FUNCTION_BLOCK FB 24
TITLE =
AUTHOR : WE_ZA
FAMILY : Ablauf
NAME : BETR
VERSION : 0.1


VAR_INPUT
  STG_AUS : BOOL ;
  STG_EIN : BOOL ;
  START : BOOL ;
  AUTO : BOOL ;
  EmB : BOOL ;
  EoB : BOOL ;
  EINR : BOOL ;
  ZYKLUS : BOOL ;
  NOT_AUS : BOOL ;
  AKTOR_FR : BOOL ;
  GST_ANL : BOOL ;
  SCHRITT : INT ;
END_VAR
VAR_OUTPUT
  ANZ_STG : BOOL ;
  ANZ_AUTO : BOOL ;
  ANZ_EmB : BOOL ;
  ANZ_EoB : BOOL ;
  ANZ_EINR : BOOL ;
  ANZ_ZYK_E : BOOL ;
  ANZ_ZYK_A : BOOL ;
  RESET : BOOL ;
  FR_K_mB : BOOL ;
  FR_K_oB : BOOL ;
  FR_AKTION : BOOL ;
END_VAR
VAR
  STEU_EIN : BOOL ;
  AUTO_EIN : BOOL ;
  AUTO_BE : BOOL ;
  START_SP : BOOL ;
  FO1 : BOOL ;
  FO2 : BOOL ;
  IO_WEITER : BOOL ;
END_VAR
BEGIN
NETWORK
TITLE =
//Steuerung EIN-AUS
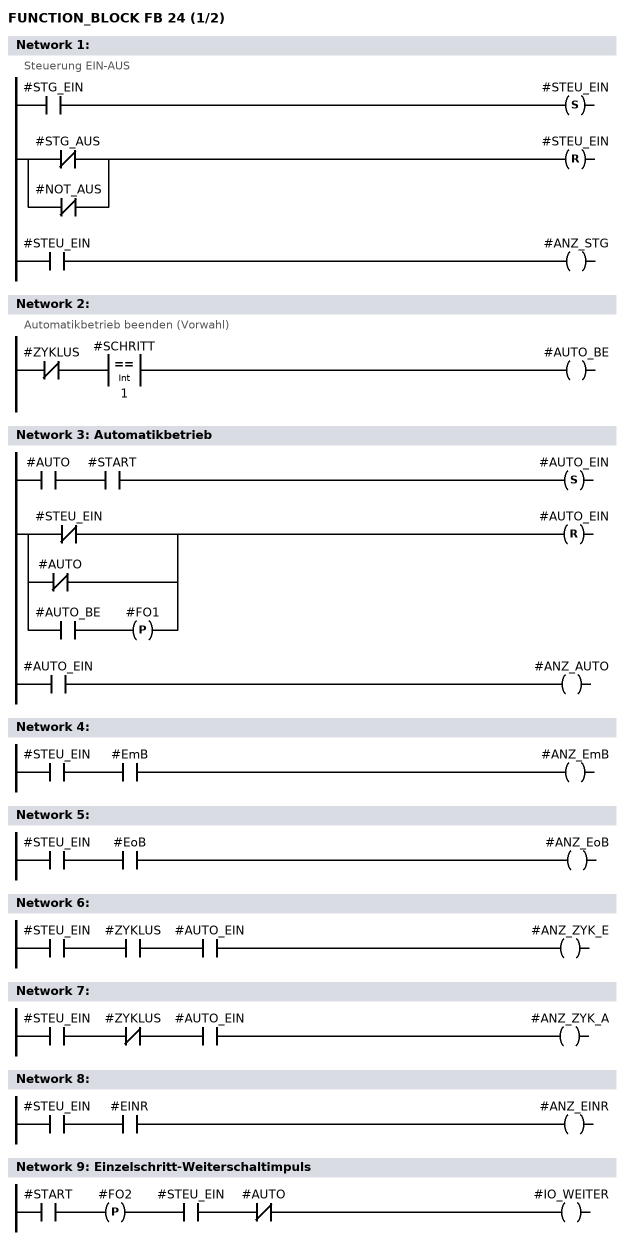
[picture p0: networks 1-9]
      U     #STG_EIN;
      S     #STEU_EIN;
      U(    ;
      ON    #STG_AUS;
      ON    #NOT_AUS;
      )     ;
      R     #STEU_EIN;
      U     #STEU_EIN;
      =     #ANZ_STG;
NETWORK
TITLE =
//Automatikbetrieb beenden (Vorwahl)
      UN    #ZYKLUS;
      U(    ;
      L     #SCHRITT;
      L     1;
      ==I   ;
      )     ;
      =     #AUTO_BE;
NETWORK
TITLE =Automatikbetrieb

      U     #AUTO;
      U     #START;
      S     #AUTO_EIN;
      U(    ;
      ON    #STEU_EIN;
      ON    #AUTO;
      O(    ;
      U     #AUTO_BE;
      FP    #FO1;
      )     ;
      )     ;
      R     #AUTO_EIN;
      U     #AUTO_EIN;
      =     #ANZ_AUTO;
NETWORK
TITLE =

      U     #STEU_EIN;
      U     #EmB;
      =     #ANZ_EmB;
NETWORK
TITLE =

      U     #STEU_EIN;
      U     #EoB;
      =     #ANZ_EoB;
NETWORK
TITLE =

      U     #STEU_EIN;
      U     #ZYKLUS;
      U     #AUTO_EIN;
      =     #ANZ_ZYK_E;
NETWORK
TITLE =

      U     #STEU_EIN;
      UN    #ZYKLUS;
      U     #AUTO_EIN;
      =     #ANZ_ZYK_A;
NETWORK
TITLE =

      U     #STEU_EIN;
      U     #EINR;
      =     #ANZ_EINR;
NETWORK
TITLE =Einzelschritt-Weiterschaltimpuls

      U     #START;
      FP    #FO2;
      U     #STEU_EIN;
      UN    #AUTO;
      =     #IO_WEITER;
NETWORK
TITLE =Freigabe Kette mit Bedingungen
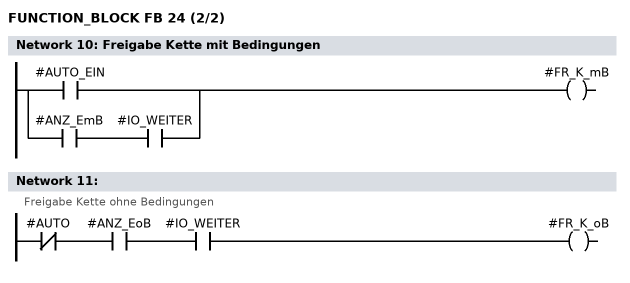
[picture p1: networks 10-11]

      O     #AUTO_EIN;
      O     ;
      U     #ANZ_EmB;
      U     #IO_WEITER;
      =     #FR_K_mB;
NETWORK
TITLE =
//Freigabe Kette ohne Bedingungen
      UN    #AUTO;
      U     #ANZ_EoB;
      U     #IO_WEITER;
      =     #FR_K_oB;
NETWORK
TITLE =Aktionsfreigabe

      U(    ;
      O     #AUTO_EIN;
      O     ;
      U     #ANZ_EmB;
      U(    ;
      U     #START;
      S     #START_SP;
      UN    #STEU_EIN;
      R     #START_SP;
      U     #START_SP;
      )     ;
      O     ;
      U     #ANZ_EoB;
      U     #AKTOR_FR;
      )     ;
      U     #STEU_EIN;
      =     #FR_AKTION;
NETWORK
TITLE =Rücksetzen Schrittkette u.a.
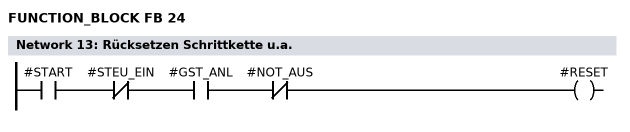
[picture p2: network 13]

      U     #START;
      UN    #STEU_EIN;
      U     #GST_ANL;
      UN    #NOT_AUS;
      =     #RESET;
END_FUNCTION_BLOCK

FUNCTION_BLOCK FB 25
TITLE =
AUTHOR : WE_ZA
FAMILY : Ablauf
NAME : KET_10
VERSION : 0.1


VAR_INPUT
  RESET : BOOL ;
  WEITER_mB : BOOL ;
  WEITER_oB : BOOL ;
  T1_2 : BOOL ;
  T2_3 : BOOL  := TRUE;
  T3_4 : BOOL  := TRUE;
  T4_5 : BOOL  := TRUE;
  T5_6 : BOOL  := TRUE;
  T6_7 : BOOL  := TRUE;
  T7_8 : BOOL  := TRUE;
  T8_9 : BOOL  := TRUE;
  T9_10 : BOOL  := TRUE;
  T10_1 : BOOL  := TRUE;
END_VAR
VAR_OUTPUT
  SCHRITT : INT ;
END_VAR
VAR
  SRO_1 : BOOL  := TRUE;
  SRO_2 : BOOL ;
  SRO_3 : BOOL ;
  SRO_4 : BOOL ;
  SRO_5 : BOOL ;
  SRO_6 : BOOL ;
  SRO_7 : BOOL ;
  SRO_8 : BOOL ;
  SRO_9 : BOOL ;
  SRO_10 : BOOL ;
END_VAR
BEGIN
NETWORK
TITLE =



      U(    ;
      U(    ;
      O     #RESET;
      O     ;
      UN    #SRO_9;
      U     #SRO_10;
      U(    ;
      U     #WEITER_mB;
      U     #T10_1;
      O     #WEITER_oB;
      )     ;
      )     ;
      S     #SRO_1;
      U     #SRO_2;
      R     #SRO_1;
      U     #SRO_1;
      )     ;
      SPBNB _001;
      L     1;
      T     #SCHRITT;
_001: NOP   0;
NETWORK
TITLE =

      U(    ;
      U     #SRO_1;
      UN    #SRO_10;
      U(    ;
      U     #WEITER_mB;
      U     #T1_2;
      O     #WEITER_oB;
      )     ;
      S     #SRO_2;
      U(    ;
      O     #RESET;
      O     #SRO_3;
      )     ;
      R     #SRO_2;
      U     #SRO_2;
      )     ;
      SPBNB _002;
      L     2;
      T     #SCHRITT;
_002: NOP   0;
NETWORK
TITLE =

      U(    ;
      U     #SRO_2;
      UN    #SRO_1;
      U(    ;
      U     #WEITER_mB;
      U     #T2_3;
      O     #WEITER_oB;
      )     ;
      S     #SRO_3;
      U(    ;
      O     #RESET;
      O     #SRO_4;
      )     ;
      R     #SRO_3;
      U     #SRO_3;
      )     ;
      SPBNB _003;
      L     3;
      T     #SCHRITT;
_003: NOP   0;
NETWORK
TITLE =

      U(    ;
      U     #SRO_3;
      UN    #SRO_2;
      U(    ;
      U     #WEITER_mB;
      U     #T3_4;
      O     #WEITER_oB;
      )     ;
      S     #SRO_4;
      U(    ;
      O     #RESET;
      O     #SRO_5;
      )     ;
      R     #SRO_4;
      U     #SRO_4;
      )     ;
      SPBNB _004;
      L     4;
      T     #SCHRITT;
_004: NOP   0;
NETWORK
TITLE =

      U(    ;
      U     #SRO_4;
      UN    #SRO_3;
      U(    ;
      U     #WEITER_mB;
      U     #T4_5;
      O     #WEITER_oB;
      )     ;
      S     #SRO_5;
      U(    ;
      O     #RESET;
      O     #SRO_6;
      )     ;
      R     #SRO_5;
      U     #SRO_5;
      )     ;
      SPBNB _005;
      L     5;
      T     #SCHRITT;
_005: NOP   0;
NETWORK
TITLE =

      U(    ;
      U     #SRO_5;
      UN    #SRO_4;
      U(    ;
      U     #WEITER_mB;
      U     #T5_6;
      O     #WEITER_oB;
      )     ;
      S     #SRO_6;
      U(    ;
      O     #RESET;
      O     #SRO_7;
      )     ;
      R     #SRO_6;
      U     #SRO_6;
      )     ;
      SPBNB _006;
      L     6;
      T     #SCHRITT;
_006: NOP   0;
NETWORK
TITLE =

      U(    ;
      U     #SRO_6;
      UN    #SRO_5;
      U(    ;
      U     #WEITER_mB;
      U     #T6_7;
      O     #WEITER_oB;
      )     ;
      S     #SRO_7;
      U(    ;
      O     #RESET;
      O     #SRO_8;
      )     ;
      R     #SRO_7;
      U     #SRO_7;
      )     ;
      SPBNB _007;
      L     7;
      T     #SCHRITT;
_007: NOP   0;
NETWORK
TITLE =

      U(    ;
      U     #SRO_7;
      UN    #SRO_6;
      U(    ;
      U     #WEITER_mB;
      U     #T7_8;
      O     #WEITER_oB;
      )     ;
      S     #SRO_8;
      U(    ;
      O     #RESET;
      O     #SRO_9;
      )     ;
      R     #SRO_8;
      U     #SRO_8;
      )     ;
      SPBNB _008;
      L     8;
      T     #SCHRITT;
_008: NOP   0;
NETWORK
TITLE =

      U(    ;
      U     #SRO_8;
      UN    #SRO_7;
      U(    ;
      U     #WEITER_mB;
      U     #T8_9;
      O     #WEITER_oB;
      )     ;
      S     #SRO_9;
      U(    ;
      O     #RESET;
      O     #SRO_10;
      )     ;
      R     #SRO_9;
      U     #SRO_9;
      )     ;
      SPBNB _009;
      L     9;
      T     #SCHRITT;
_009: NOP   0;
NETWORK
TITLE =

      U(    ;
      U     #SRO_9;
      UN    #SRO_8;
      U(    ;
      U     #WEITER_mB;
      U     #T9_10;
      O     #WEITER_oB;
      )     ;
      S     #SRO_10;
      U(    ;
      O     #RESET;
      O     #SRO_1;
      )     ;
      R     #SRO_10;
      U     #SRO_10;
      )     ;
      SPBNB _00a;
      L     10;
      T     #SCHRITT;
_00a: NOP   0;
END_FUNCTION_BLOCK

FUNCTION FC 26 : VOID
TITLE =
VERSION : 0.1


VAR_INPUT
  SCHRITT : INT ;
  FREIGABE : BOOL ;
  EINRI : BOOL ;
  RESET : BOOL ;
  A_ANW : BYTE ;
  A_AST : BOOL ;
  A_GST : BOOL ;
  _1B1 : BOOL ;
  _1B2 : BOOL ;
  _2B1 : BOOL ;
  _3B1 : BOOL ;
  S1 : BOOL ;
  S2 : BOOL ;
  S3 : BOOL ;
  Zeit_1 : TIMER ;
  Zeitw_1 : S5TIME ;
  Zeit_2 : TIMER ;
  Zeitw_2 : S5TIME ;
END_VAR
VAR_OUTPUT
  _1Y1 : BOOL ;
  _1Y2 : BOOL ;
  _2Y1 : BOOL ;
  _3Y1 : BOOL ;
  K1 : BOOL ;
  K2 : BOOL ;
END_VAR
VAR_TEMP
  Aktor : INT ;
END_VAR
BEGIN
NETWORK
TITLE =

      L     #A_ANW;
      L     B#16#F;
      UW    ;
      T     #Aktor;
NETWORK
TITLE =Ansteuerung 1Y1 Zylinder 1A vor
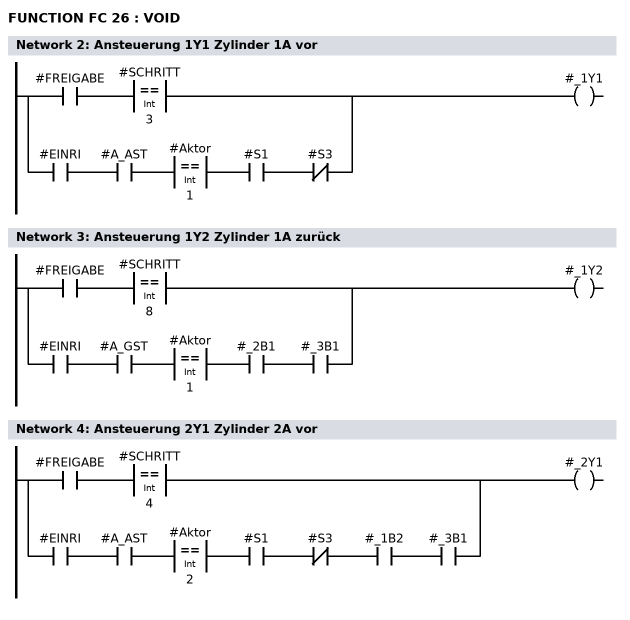
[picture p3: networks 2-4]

      U     #FREIGABE;
      U(    ;
      L     #SCHRITT;
      L     3;
      ==I   ;
      )     ;
      O     ;
      U     #EINRI;
      U     #A_AST;
      U(    ;
      L     #Aktor;
      L     1;
      ==I   ;
      )     ;
      U     #S1;
      UN    #S3;
      =     #_1Y1;
NETWORK
TITLE =Ansteuerung 1Y2 Zylinder 1A zurück

      U     #FREIGABE;
      U(    ;
      L     #SCHRITT;
      L     8;
      ==I   ;
      )     ;
      O     ;
      U     #EINRI;
      U     #A_GST;
      U(    ;
      L     #Aktor;
      L     1;
      ==I   ;
      )     ;
      U     #_2B1;
      U     #_3B1;
      =     #_1Y2;
NETWORK
TITLE =Ansteuerung 2Y1 Zylinder 2A vor

      U     #FREIGABE;
      U(    ;
      L     #SCHRITT;
      L     4;
      ==I   ;
      )     ;
      O     ;
      U     #EINRI;
      U     #A_AST;
      U(    ;
      L     #Aktor;
      L     2;
      ==I   ;
      )     ;
      U     #S1;
      UN    #S3;
      U     #_1B2;
      U     #_3B1;
      =     #_2Y1;
NETWORK
TITLE =Ansteuerung 2Y1 Zylinder 3A vor

      U     #FREIGABE;
      U(    ;
      O(    ;
      L     #SCHRITT;
      L     6;
      ==I   ;
      )     ;
      O(    ;
      U(    ;
      L     #SCHRITT;
      L     7;
      ==I   ;
      )     ;
      L     #Zeitw_1;
      SI    #Zeit_1;
      U(    ;
      O     #RESET;
      ON    #FREIGABE;
      )     ;
      R     #Zeit_1;
      NOP   0;
      NOP   0;
      U     #Zeit_1;
      )     ;
      )     ;
      O     ;
      U     #EINRI;
      U     #A_AST;
      U(    ;
      L     #Aktor;
      L     3;
      ==I   ;
      )     ;
      U     #S1;
      UN    #S3;
      U     #_1B2;
      U     #_2B1;
      =     #_3Y1;
NETWORK
TITLE = Ansteuerung K1 Schutztür zu

      U(    ;
      U     #FREIGABE;
      U(    ;
      U(    ;
      L     #SCHRITT;
      L     2;
      ==I   ;
      )     ;
      L     #Zeitw_2;
      SE    #Zeit_2;
      U(    ;
      O     #RESET;
      ON    #FREIGABE;
      )     ;
      R     #Zeit_2;
      NOP   0;
      NOP   0;
      U     #Zeit_2;
      )     ;
      O     ;
      U     #EINRI;
      U     #A_AST;
      U(    ;
      L     #Aktor;
      L     4;
      ==I   ;
      )     ;
      )     ;
      U     #S3;
      =     #K1;
NETWORK
TITLE =Ansteuerung K2 Schutztüre Auf
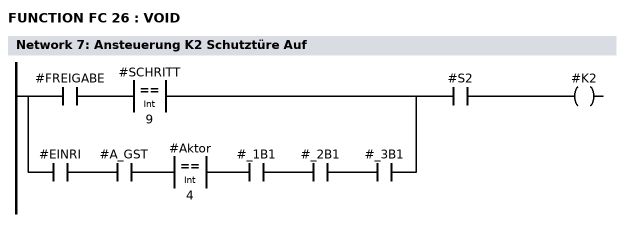
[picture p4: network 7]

      U(    ;
      U     #FREIGABE;
      U(    ;
      L     #SCHRITT;
      L     9;
      ==I   ;
      )     ;
      O     ;
      U     #EINRI;
      U     #A_GST;
      U(    ;
      L     #Aktor;
      L     4;
      ==I   ;
      )     ;
      U     #_1B1;
      U     #_2B1;
      U     #_3B1;
      )     ;
      U     #S2;
      =     #K2;
END_FUNCTION

ORGANIZATION_BLOCK OB 1
TITLE = "Main Program Sweep (Cycle)"
VERSION : 0.1


VAR_TEMP
  OB1_EV_CLASS : BYTE ;	//Bits 0-3 = 1 (Coming event), Bits 4-7 = 1 (Event class 1)
  OB1_SCAN_1 : BYTE ;	//1 (Cold restart scan 1 of OB 1), 3 (Scan 2-n of OB 1)
  OB1_PRIORITY : BYTE ;	//Priority of OB Execution
  OB1_OB_NUMBR : BYTE ;	//1 (Organization block 1, OB1)
  OB1_RESERVED_1 : BYTE ;	//Reserved for system
  OB1_RESERVED_2 : BYTE ;	//Reserved for system
  OB1_PREV_CYCLE : INT ;	//Cycle time of previous OB1 scan (milliseconds)
  OB1_MIN_CYCLE : INT ;	//Minimum cycle time of OB1 (milliseconds)
  OB1_MAX_CYCLE : INT ;	//Maximum cycle time of OB1 (milliseconds)
  OB1_DATE_TIME : DATE_AND_TIME ;	//Date and time OB1 started
  GA : BOOL ;
  Schritt : INT ;
  B0 : BOOL ;
  B1 : BOOL ;
  B2 : BOOL ;
  B3 : BOOL ;
END_VAR
BEGIN
NETWORK
TITLE =
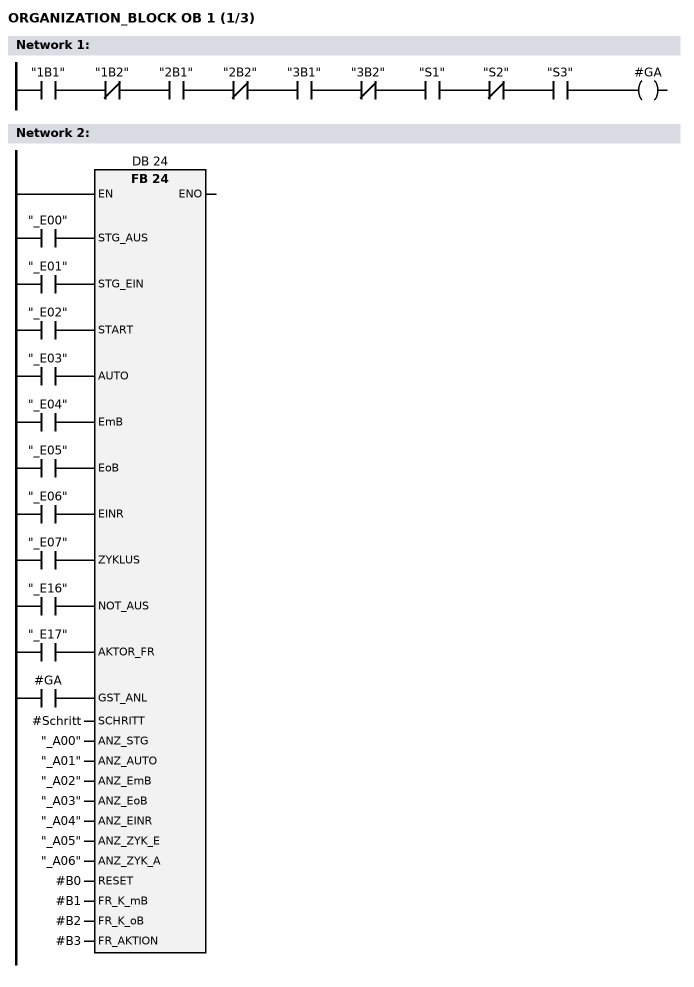
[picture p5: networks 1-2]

      U     "1B1";
      UN    "1B2";
      U     "2B1";
      UN    "2B2";
      U     "3B1";
      UN    "3B2";
      U     "S1";
      UN    "S2";
      U     "S3";
      =     #GA;
NETWORK
TITLE =

      U     "_E00";
      =     L     25.0;
      BLD   103;
      U     "_E01";
      =     L     25.1;
      BLD   103;
      U     "_E02";
      =     L     25.2;
      BLD   103;
      U     "_E03";
      =     L     25.3;
      BLD   103;
      U     "_E04";
      =     L     25.4;
      BLD   103;
      U     "_E05";
      =     L     25.5;
      BLD   103;
      U     "_E06";
      =     L     25.6;
      BLD   103;
      U     "_E07";
      =     L     25.7;
      BLD   103;
      U     "_E16";
      =     L     26.0;
      BLD   103;
      U     "_E17";
      =     L     26.1;
      BLD   103;
      U     #GA;
      =     L     26.2;
      BLD   103;
      CALL FB    24 , DB    24 (
           STG_AUS                  := L     25.0,
           STG_EIN                  := L     25.1,
           START                    := L     25.2,
           AUTO                     := L     25.3,
           EmB                      := L     25.4,
           EoB                      := L     25.5,
           EINR                     := L     25.6,
           ZYKLUS                   := L     25.7,
           NOT_AUS                  := L     26.0,
           AKTOR_FR                 := L     26.1,
           GST_ANL                  := L     26.2,
           SCHRITT                  := #Schritt,
           ANZ_STG                  := "_A00",
           ANZ_AUTO                 := "_A01",
           ANZ_EmB                  := "_A02",
           ANZ_EoB                  := "_A03",
           ANZ_EINR                 := "_A04",
           ANZ_ZYK_E                := "_A05",
           ANZ_ZYK_A                := "_A06",
           RESET                    := #B0,
           FR_K_mB                  := #B1,
           FR_K_oB                  := #B2,
           FR_AKTION                := #B3);
      NOP   0;
NETWORK
TITLE =
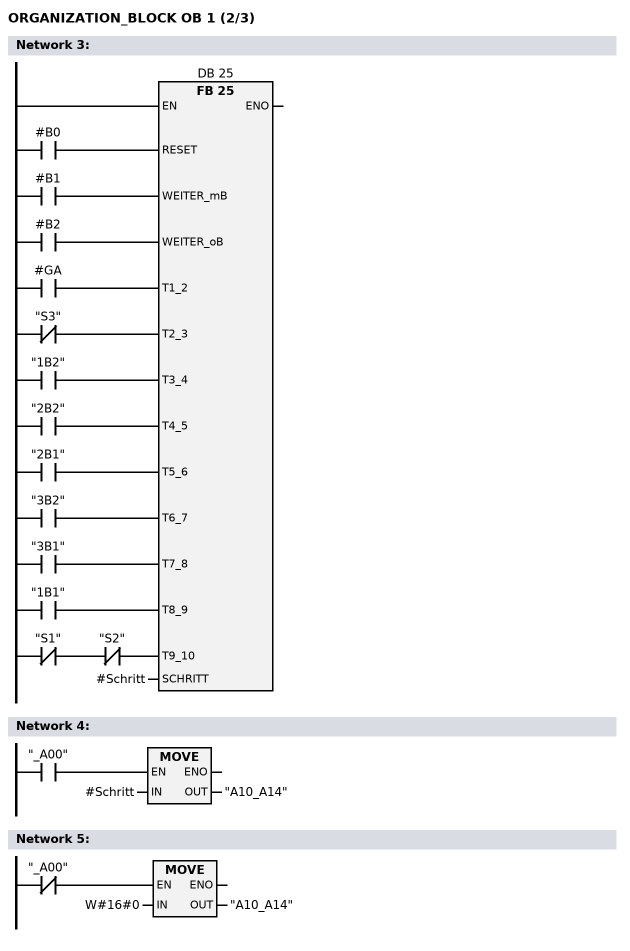
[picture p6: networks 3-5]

      U     #B0;
      =     L     25.0;
      BLD   103;
      U     #B1;
      =     L     25.1;
      BLD   103;
      U     #B2;
      =     L     25.2;
      BLD   103;
      U     #GA;
      =     L     25.3;
      BLD   103;
      UN    "S3";
      =     L     25.4;
      BLD   103;
      U     "1B2";
      =     L     25.5;
      BLD   103;
      U     "2B2";
      =     L     25.6;
      BLD   103;
      U     "2B1";
      =     L     25.7;
      BLD   103;
      U     "3B2";
      =     L     26.0;
      BLD   103;
      U     "3B1";
      =     L     26.1;
      BLD   103;
      U     "1B1";
      =     L     26.2;
      BLD   103;
      UN    "S1";
      UN    "S2";
      =     L     26.3;
      BLD   103;
      CALL FB    25 , DB    25 (
           RESET                    := L     25.0,
           WEITER_mB                := L     25.1,
           WEITER_oB                := L     25.2,
           T1_2                     := L     25.3,
           T2_3                     := L     25.4,
           T3_4                     := L     25.5,
           T4_5                     := L     25.6,
           T5_6                     := L     25.7,
           T6_7                     := L     26.0,
           T7_8                     := L     26.1,
           T8_9                     := L     26.2,
           T9_10                    := L     26.3,
           SCHRITT                  := #Schritt);
      NOP   0;
NETWORK
TITLE =

      U     "_A00";
      SPBNB _001;
      L     #Schritt;
      T     "A10_A14";
_001: NOP   0;
NETWORK
TITLE =

      UN    "_A00";
      SPBNB _002;
      L     W#16#0;
      T     "A10_A14";
_002: NOP   0;
NETWORK
TITLE =Ausgabebaustein
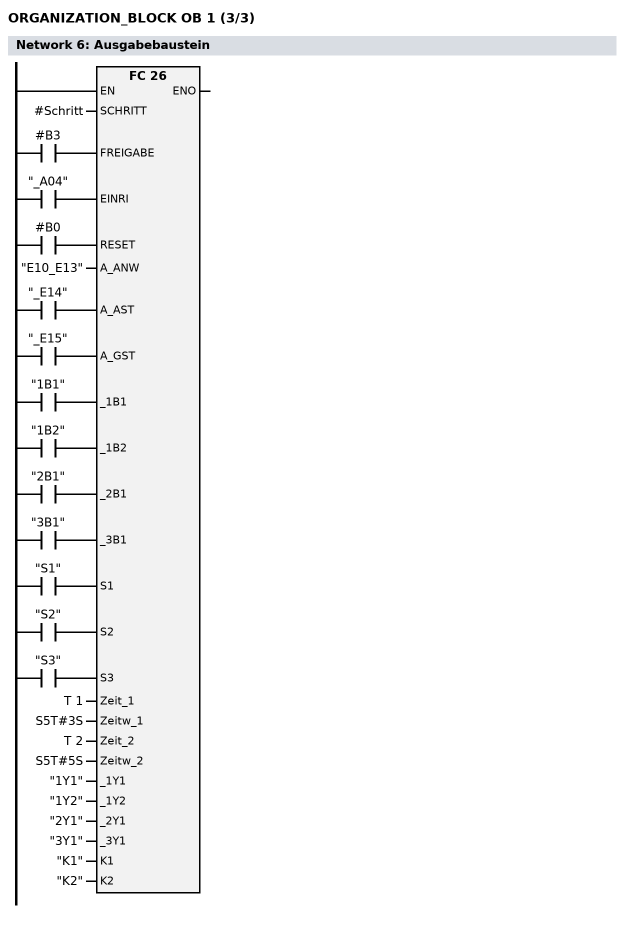
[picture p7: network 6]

      U     #B3;
      =     L     25.0;
      BLD   103;
      U     "_A04";
      =     L     25.1;
      BLD   103;
      U     #B0;
      =     L     25.2;
      BLD   103;
      U     "_E14";
      =     L     25.3;
      BLD   103;
      U     "_E15";
      =     L     25.4;
      BLD   103;
      U     "1B1";
      =     L     25.5;
      BLD   103;
      U     "1B2";
      =     L     25.6;
      BLD   103;
      U     "2B1";
      =     L     25.7;
      BLD   103;
      U     "3B1";
      =     L     26.0;
      BLD   103;
      U     "S1";
      =     L     26.1;
      BLD   103;
      U     "S2";
      =     L     26.2;
      BLD   103;
      U     "S3";
      =     L     26.3;
      BLD   103;
      CALL FC    26 (
           SCHRITT                  := #Schritt,
           FREIGABE                 := L     25.0,
           EINRI                    := L     25.1,
           RESET                    := L     25.2,
           A_ANW                    := "E10_E13",
           A_AST                    := L     25.3,
           A_GST                    := L     25.4,
           _1B1                     := L     25.5,
           _1B2                     := L     25.6,
           _2B1                     := L     25.7,
           _3B1                     := L     26.0,
           S1                       := L     26.1,
           S2                       := L     26.2,
           S3                       := L     26.3,
           Zeit_1                   := T      1,
           Zeitw_1                  := S5T#3S,
           Zeit_2                   := T      2,
           Zeitw_2                  := S5T#5S,
           _1Y1                     := "1Y1",
           _1Y2                     := "1Y2",
           _2Y1                     := "2Y1",
           _3Y1                     := "3Y1",
           K1                       := "K1",
           K2                       := "K2");
      NOP   0;
END_ORGANIZATION_BLOCK

ORGANIZATION_BLOCK OB 2
TITLE =
VERSION : 0.1


VAR_TEMP
  Default : ARRAY  [1 .. 20 ] OF BYTE ;
  Schritt : INT ;
  B0 : BOOL ;
  B1 : BOOL ;
  B2 : BOOL ;
  B3 : BOOL ;
  GA : BOOL ;
END_VAR
BEGIN
NETWORK
TITLE =
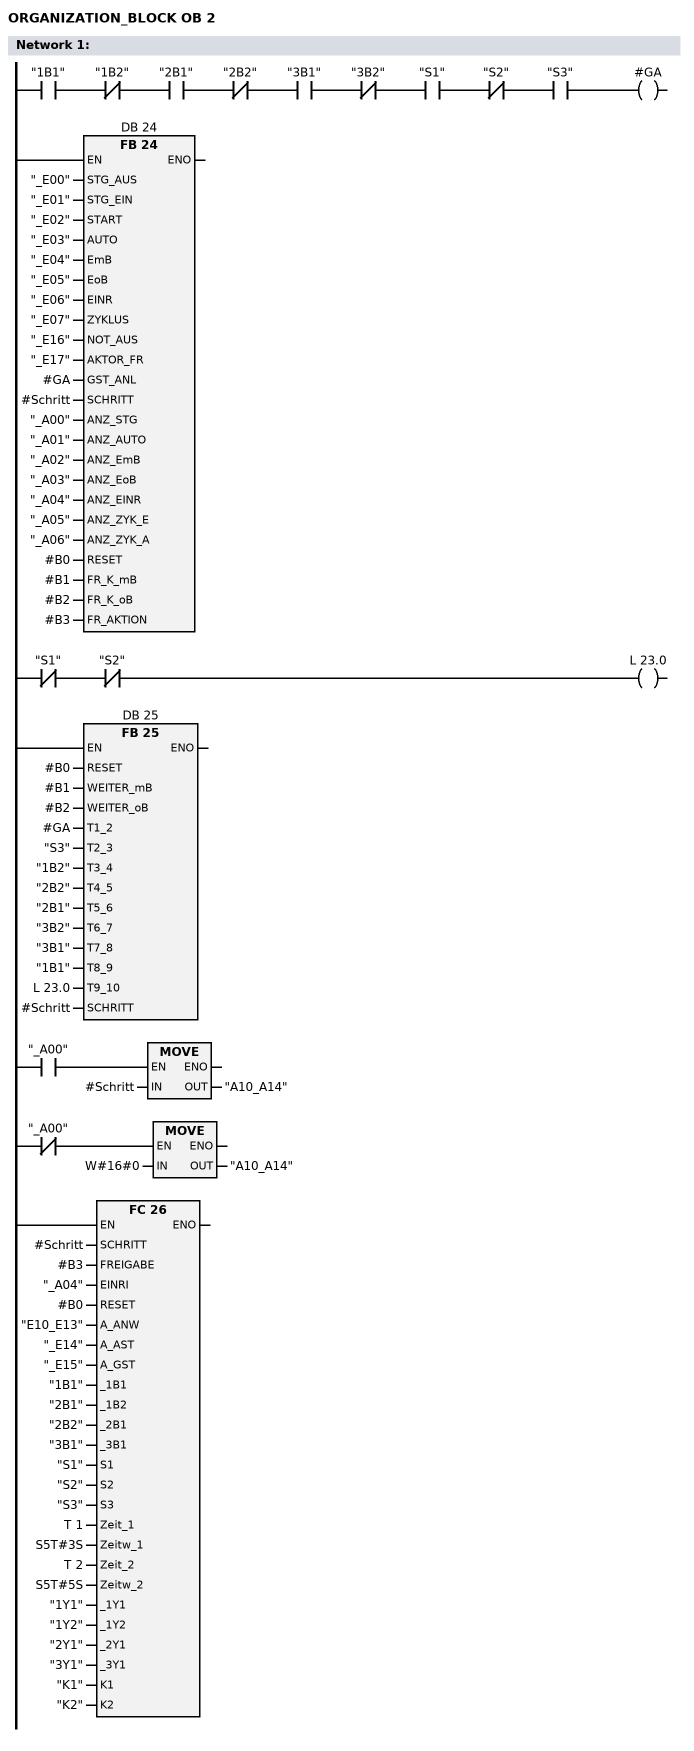
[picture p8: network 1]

      U     "1B1";
      UN    "1B2";
      U     "2B1";
      UN    "2B2";
      U     "3B1";
      UN    "3B2";
      U     "S1";
      UN    "S2";
      U     "S3";
      =     #GA;
      CALL FB    24 , DB    24 (
           STG_AUS                  := "_E00",
           STG_EIN                  := "_E01",
           START                    := "_E02",
           AUTO                     := "_E03",
           EmB                      := "_E04",
           EoB                      := "_E05",
           EINR                     := "_E06",
           ZYKLUS                   := "_E07",
           NOT_AUS                  := "_E16",
           AKTOR_FR                 := "_E17",
           GST_ANL                  := #GA,
           SCHRITT                  := #Schritt,
           ANZ_STG                  := "_A00",
           ANZ_AUTO                 := "_A01",
           ANZ_EmB                  := "_A02",
           ANZ_EoB                  := "_A03",
           ANZ_EINR                 := "_A04",
           ANZ_ZYK_E                := "_A05",
           ANZ_ZYK_A                := "_A06",
           RESET                    := #B0,
           FR_K_mB                  := #B1,
           FR_K_oB                  := #B2,
           FR_AKTION                := #B3);

      UN    "S1";
      UN    "S2";
      =     L     23.0;

      CALL FB    25 , DB    25 (
           RESET                    := #B0,
           WEITER_mB                := #B1,
           WEITER_oB                := #B2,
           T1_2                     := #GA,
           T2_3                     := "S3",
           T3_4                     := "1B2",
           T4_5                     := "2B2",
           T5_6                     := "2B1",
           T6_7                     := "3B2",
           T7_8                     := "3B1",
           T8_9                     := "1B1",
           T9_10                    := L     23.0,
           SCHRITT                  := #Schritt);


      U     "_A00";
      SPBNB _001;
      L     #Schritt;
      T     "A10_A14";
_001: NOP   0;

      UN    "_A00";
      SPBNB _002;
      L     W#16#0;
      T     "A10_A14";
_002: NOP   0;




      CALL FC    26 (
           SCHRITT                  := #Schritt,
           FREIGABE                 := #B3,
           EINRI                    := "_A04",
           RESET                    := #B0,
           A_ANW                    := "E10_E13",
           A_AST                    := "_E14",
           A_GST                    := "_E15",
           _1B1                     := "1B1",
           _1B2                     := "2B1",
           _2B1                     := "2B2",
           _3B1                     := "3B1",
           S1                       := "S1",
           S2                       := "S2",
           S3                       := "S3",
           Zeit_1                   := T      1,
           Zeitw_1                  := S5T#3S,
           Zeit_2                   := T      2,
           Zeitw_2                  := S5T#5S,
           _1Y1                     := "1Y1",
           _1Y2                     := "1Y2",
           _2Y1                     := "2Y1",
           _3Y1                     := "3Y1",
           K1                       := "K1",
           K2                       := "K2");
      NOP   0;

END_ORGANIZATION_BLOCK

